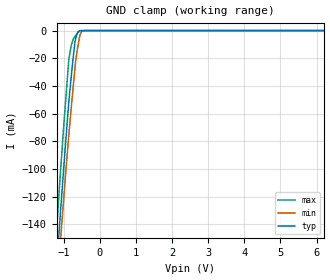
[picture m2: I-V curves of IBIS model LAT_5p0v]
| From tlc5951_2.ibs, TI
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|   lat_5p0v Model
[Model]   LAT_5p0v
Model_type   Input
Vinl = 1.5
Vinh = 3.5
|   typ   min   max
|   (nom PVT)   (Fast PVT)   (slow PVT)
|Average
C_comp   1.182e-12   1.169e-12   1.285e-12
| Where nom  PVT is Nominal Process,  5V,  65C
|   Fast PVT is Strong Process,   5.5V,  -40C
|   Slow PVT is Weak Process,   4.5V,  125C
[Model Spec]
Vinl   1.5   1.35   1.65
Vinh   3.5   3.15   3.85
[Voltage Range]   5   4.5   5.5
|Ambient Temperature   25   85   -40
|Junction Temperature
[Temperature Range]   65   125   -40
[Power Clamp Reference]   5   4.5   5.5
[GND Clamp Reference]   0   0   0
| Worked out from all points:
|   GND clamp passes 1 mA (typ) near -0.61 V on its own axis
[GND Clamp]
|   Voltage   I(typ)   I(min)   I(max)
-5V       -1.792A    -1.69A     -1.896A
-1.255V   -192.8mA   -209.7mA   -169.1mA
-1.139V   -149mA     -168.6mA   -120.7mA
-1.085V   -129.2mA   -149.8mA   -100mA
-1.007V   -101.6mA   -123.6mA   -71.23mA
-853mV    -49.49mA   -73.69mA   -19.85mA
-787mV    -31.88mA   -54.21mA   -10.18mA
-690mV    -8.341mA   -27.32mA   -4.319mA
-615mV    -1.319mA   -12.25mA   -1.719mA
-549.5mV  -21.76uA   -3.216mA   -238.5uA
-414.5mV  0A         0A         0A
10V       0A         0A         0A
[POWER Clamp]
|   Voltage   I(typ)   I(min)   I(max)
-5V       0A         0A         0A
10V       0A         0A         0A
